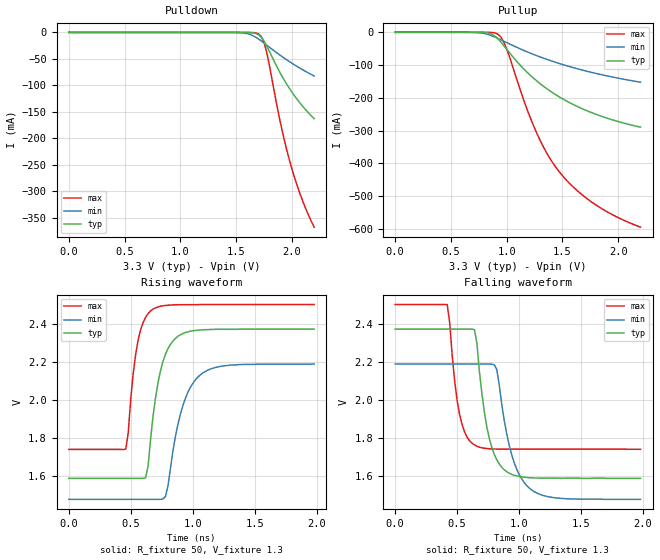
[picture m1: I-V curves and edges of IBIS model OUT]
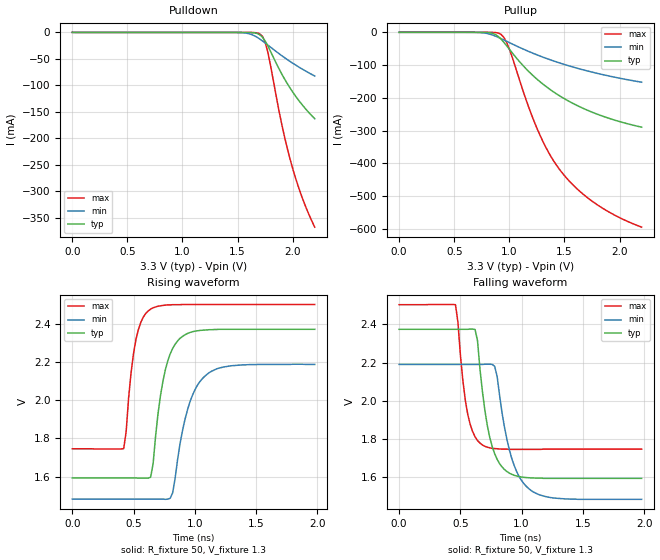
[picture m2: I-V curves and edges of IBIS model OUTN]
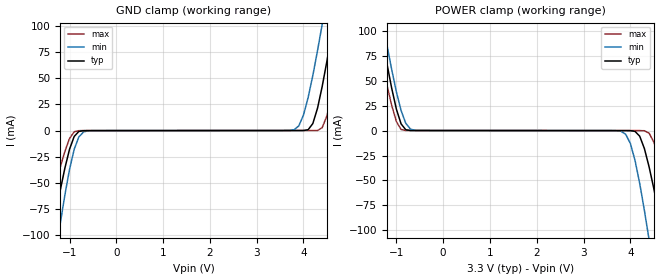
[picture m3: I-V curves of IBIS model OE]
[IBIS Ver]   3.2
[Comment Char]   |_char
[File name]   vg4513ca.ibs
[File Rev]   1.0
[Date]   2014/07/30 8:52:33
[Source]
[Notes]
[Disclaimer]
Seiko Epson Corporation makes no warranty with respect to the information
contained herein.
[Copyright]
Copyright(C) 2014, Seiko Epson Corporation. All rights reserved.
[Component]   vg4513ca
Si_location Pin
Timing_location Pin
[Manufacturer]   Seiko Epson Corporation
[Package]
R_pkg   0.36   NA   NA
L_pkg   4.00n   NA   NA
C_pkg   0.70p   NA   NA
[Pin] signal_name   model_name   R_pin   L_pin   C_pin
1   VC   NC
2   OE   OE   0.10   2.00n   1.74p
3   GND   GND
4   OUT   OUT   0.43   4.00n   0.90p
5   OUTN   OUTN   0.28   4.00n   0.51p
6   VCC   POWER
[Diff Pin] inv_pin vdiff   tdelay_typ
4   5   0   0
| Models and submodels in the file (3): OUT (Output_ECL), OUTN (Output_ECL), OE (Input)
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[Model]   OUT
Model_type Output_ECL
Enable Active-High
Polarity Non-Inverting
Vref=1.3
Vmeas=1.982
Rref=50
Cref=0
C_comp   0.1p   0.1p   0.1p
[Temperature Range] 25   110   -40
[Voltage Range]   3.3   3.135   3.465
[Pullup Reference]  3.3   3.135   3.465
[Pulldown Reference]3.3   3.135   3.465
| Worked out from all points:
|   falling waveform, R_fixture 50, V_fixture 1.3: 20-80 % time 112ps typ, 146ps min, 84.8ps max; typ from 2.37 V to 1.59 V
|   rising waveform, R_fixture 50, V_fixture 1.3: 20-80 % time 114ps typ, 150ps min, 85.1ps max; typ from 1.59 V to 2.37 V
[Pullup]
0V        109.6pA    1.947nA    59.12pA
800mV     -591.5uA   -3.656mA   -20.64uA
875mV     -6.95mA    -11.77mA   -732.2uA
925mV     -20.96mA   -19.23mA   -6.473mA
1V        -51.65mA   -31.36mA   -50.91mA
1.15V     -110.7mA   -54.7mA    -204.2mA
1.25V     -142.7mA   -68.65mA   -292.4mA
1.35V     -169.6mA   -81.31mA   -362.8mA
1.45V     -192.5mA   -92.77mA   -415.9mA
1.6V      -220.8mA   -108mA     -472.9mA
1.775V    -246.8mA   -123.4mA   -520.8mA
2.2V      -289.3mA   -152.1mA   -594.3mA
[Pulldown]
0V        122.4uA    211.1uA    4.794uA
1.525V    -7.282uA   -320.5uA   -606.9nA
1.625V    -306uA     -3.796mA   -71.84uA
1.7V      -4.268mA   -12.26mA   -2.476mA
1.725V    -8.871mA   -15.98mA   -7.297mA
1.75V     -16.14mA   -19.91mA   -18.42mA
1.775V    -25.6mA    -23.95mA   -37.74mA
1.9V      -78.19mA   -43.75mA   -172.8mA
1.95V     -96.31mA   -51.08mA   -218.2mA
2V        -112.5mA   -58.03mA   -257.1mA
2.1V      -140.1mA   -70.8mA    -319.6mA
2.2V      -162.9mA   -82.28mA   -367.6mA
[Falling Waveform]
R_fixture=50
V_fixture=1.3
V_fixture_min=1.135
V_fixture_max=1.465
0s        2.371V     2.188V     2.5V
420ps     2.371V     2.188V     2.499V
520ps     2.371V     2.188V     1.922V
640ps     2.368V     2.188V     1.764V
740ps     1.857V     2.188V     1.745V
820ps     1.686V     2.159V     1.742V
880ps     1.634V     1.892V     1.742V
980ps     1.602V     1.638V     1.742V
1.12ns    1.591V     1.52V      1.742V
1.98ns    1.589V     1.479V     1.741V
[Rising Waveform]
R_fixture=50
V_fixture=1.3
V_fixture_min=1.135
V_fixture_max=1.465
0s        1.59V      1.48V      1.742V
460ps     1.59V      1.48V      1.744V
560ps     1.59V      1.48V      2.317V
620ps     1.593V     1.48V      2.435V
680ps     1.917V     1.48V      2.478V
740ps     2.154V     1.48V      2.493V
800ps     2.27V      1.549V     2.498V
920ps     2.349V     1.97V      2.501V
1.06ns    2.368V     2.132V     2.502V
1.98ns    2.373V     2.19V      2.502V
[Ramp]
R_load=50
dV/dt_r   4.702e-1/1.133e-10   4.262e-1/1.496e-10   4.568e-1/8.476e-11
dV/dt_f   4.702e-1/1.119e-10   4.262e-1/1.458e-10   4.568e-1/8.461e-11
|[End   OUT
[Model]   OUTN
Model_type Output_ECL
Enable Active-High
Polarity Inverting
Vref=1.3
Vmeas=1.981
Rref=50
Cref=0
C_comp   0.1p   0.1p   0.1p
[Model Spec]
[Temperature Range] 25   110   -40
[Voltage Range]   3.3   3.135   3.465
[Pullup Reference]  3.3   3.135   3.465
[Pulldown Reference]3.3   3.135   3.465
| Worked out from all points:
|   falling waveform, R_fixture 50, V_fixture 1.3: 20-80 % time 112ps typ, 147ps min, 84.9ps max; typ from 2.37 V to 1.59 V
|   rising waveform, R_fixture 50, V_fixture 1.3: 20-80 % time 114ps typ, 149ps min, 85.3ps max; typ from 1.59 V to 2.37 V
[Pullup]
0V        109.6pA    1.951nA    59.12pA
800mV     -591.1uA   -3.655mA   -20.65uA
875mV     -6.947mA   -11.77mA   -732.3uA
925mV     -20.95mA   -19.23mA   -6.474mA
1V        -51.64mA   -31.35mA   -50.92mA
1.15V     -110.7mA   -54.69mA   -204.2mA
1.25V     -142.7mA   -68.65mA   -292.4mA
1.35V     -169.6mA   -81.3mA    -362.8mA
1.45V     -192.5mA   -92.77mA   -415.9mA
1.6V      -220.8mA   -108mA     -472.9mA
1.775V    -246.8mA   -123.3mA   -520.8mA
2.2V      -289.3mA   -152.1mA   -594.3mA
[Pulldown]
0V        122.4uA    211.1uA    4.795uA
1.525V    -7.286uA   -320.7uA   -606.7nA
1.625V    -306.2uA   -3.798mA   -71.83uA
1.7V      -4.27mA    -12.26mA   -2.475mA
1.725V    -8.875mA   -15.98mA   -7.296mA
1.75V     -16.14mA   -19.91mA   -18.42mA
1.775V    -25.6mA    -23.95mA   -37.74mA
1.9V      -78.2mA    -43.75mA   -172.8mA
1.95V     -96.32mA   -51.09mA   -218.2mA
2V        -112.5mA   -58.03mA   -257.1mA
2.1V      -140.1mA   -70.8mA    -319.6mA
2.2V      -162.9mA   -82.28mA   -367.6mA
[Falling Waveform]
R_fixture=50
V_fixture=1.3
V_fixture_min=1.135
V_fixture_max=1.465
0s        2.374V     2.19V      2.503V
460ps     2.374V     2.19V      2.503V
560ps     2.374V     2.19V      1.929V
620ps     2.373V     2.19V      1.811V
680ps     2.048V     2.19V      1.768V
740ps     1.807V     2.191V     1.753V
800ps     1.693V     2.127V     1.748V
920ps     1.614V     1.696V     1.745V
1.06ns    1.596V     1.538V     1.745V
1.98ns    1.593V     1.483V     1.746V
[Rising Waveform]
R_fixture=50
V_fixture=1.3
V_fixture_min=1.135
V_fixture_max=1.465
0s        1.593V     1.482V     1.746V
420ps     1.593V     1.482V     1.747V
520ps     1.593V     1.482V     2.319V
640ps     1.597V     1.482V     2.478V
760ps     2.16V      1.481V     2.499V
820ps     2.272V     1.516V     2.501V
880ps     2.325V     1.773V     2.501V
980ps     2.359V     2.024V     2.502V
1.12ns    2.37V      2.146V     2.502V
1.98ns    2.372V     2.188V     2.502V
[Ramp]
R_load=50
dV/dt_r   4.696E-1/1.143E-10   4.255E-1/1.506E-10   4.556E-1/8.547E-11
dV/dt_f   4.696E-1/1.127E-10   4.255E-1/1.472E-10   4.556E-1/8.522E-11
|[End   OUTN
[Model]   OE
Model_type Input
Vinh=2.2
Vinl=1.8
C_comp   2p   2p   2p
[Model Spec]
[Temperature Range] 25   110   -40
[Voltage Range]   3.3   3.135   3.465
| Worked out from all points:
|   GND clamp passes 1 mA (typ) near -0.80 V on its own axis
|   POWER clamp passes 1 mA (typ) near -0.80 V on its own axis
[GND Clamp]
-3.3V     -614.5mA   -809.6mA   -431.2mA
-1.6V     -156mA     -216mA     -106mA
-1.4V     -105.4mA   -151mA     -69.78mA
-1.2V     -57.78mA   -89.94mA   -35.51mA
-900mV    -5.677mA   -17.99mA   -1.153mA
-600mV    -82.32uA   -224.5uA   -82.43uA
3.8V      10.34uA    681.1uA    6.789uA
4V        41.56uA    14.86mA    10.84uA
4.3V      21.39mA    76.59mA    91.28uA
4.6V      92.16mA    155.3mA    31.83mA
4.9V      174.6mA    239.2mA    97.17mA
6.6V      675.5mA    740.7mA    510.3mA
[POWER Clamp]
-3.3V     675.5mA    691.2mA    551.1mA
-1.5V     146.6mA    164.9mA    112.2mA
-1.3V     92.16mA    111mA      66.64mA
-900mV    6.691mA    20.13mA    1.004mA
-600mV    13.02uA    143.3uA    12.16uA
3.8V      -78.6uA    -711.9uA   -77.01uA
4V        -124.1uA   -12.89mA   -81.08uA
4.3V      -18.02mA   -79.91mA   -210.9uA
4.4V      -36.28mA   -109.2mA   -2.598mA
4.7V      -105.4mA   -204.4mA   -41.26mA
5.1V      -208.2mA   -339.4mA   -112.5mA
6.6V      -614.5mA   -868.6mA   -399.1mA
